|   IBIS file stm32l471_476_486_lqfp144.ibs
[IBIS ver]   4.2
[File name]   stm32l471_476_486_lqfp144.ibs
[File Rev]   4.0
[Date]   05-10-2018
[Source]   Data Created at STMicroelectronics
[Notes]   File originated from ELDO simulations.
[Disclaimer]  This information is for modeling purpose only and is
   not guaranteed.
   The information is subject to change without notice.
[Copyright]   Copyright 2018 STMicroelectronics Inc.
|   Component stm32l471_476_486_lqfp144
[Component] stm32l471_476_486_lqfp144
[Manufacturer] STMicroelectronics
[Package]
| variable   typ   min   max
R_pkg   0.0   0.0   0.0
L_pkg   0.0H   0.0H   0.0H
C_pkg   0.0F   0.0F   0.0F
[Pin]  signal_name   model_name   R_pin   L_pin   C_pin
1 PE2 io8prog2m25m50m120m_sudq_ft 187.6E-3 9.4E-9 267.9E-15
2 PE3 io8prog2m25m50m120m_sudq_ft 182.4E-3 9.1E-9 243.8E-15
3 PE4 io8prog2m25m50m120m_sudq_ft 177.6E-3 8.7E-9 221.3E-15
4 PE5 io8prog2m25m50m120m_sudq_ft 173.1E-3 8.4E-9 200.2E-15
5 PE6 io8prog2m25m50m120m_sudq_ft 168.9E-3 8.1E-9 180.5E-15
6 VBAT POWER 165.0E-3 7.8E-9 162.3E-15
7 PC13 io8prog2m25m50m120m_sudq_ft 161.5E-3 7.6E-9 145.6E-15
8 PC14-OSC32_IN io8prog2m25m50m120m_sudq_ft 158.2E-3 7.4E-9 130.3E-15
9 PC15-OSC32_OUT io8prog2m25m50m120m_sudq_ft 155.2E-3 7.2E-9 116.4E-15
10 PF0 io8prog2m25m50m120m_sudq_i2c_ft 152.6E-3 7.0E-9 104.1E-15
11 PF1 io8prog2m25m50m120m_sudq_i2c_ft 150.3E-3 6.8E-9 93.2E-15
12 PF2 io8prog2m25m50m120m_sudq_ft 148.2E-3 6.7E-9 83.7E-15
13 PF3 io8prog2m25m50m120m_sudq_ft 146.5E-3 6.5E-9 75.7E-15
14 PF4 io8prog2m25m50m120m_sudq_ft 145.1E-3 6.4E-9 69.1E-15
15 PF5 io8prog2m25m50m120m_sudq_ft 144.1E-3 6.4E-9 64.0E-15
16 VSS GND 143.3E-3 6.3E-9 60.4E-15
17 VDD POWER 142.8E-3 6.3E-9 58.2E-15
18 PF6 io8prog2m25m50m120m_sudq_ft 142.7E-3 6.3E-9 57.5E-15
19 PF7 io8prog2m25m50m120m_sudq_ft 142.7E-3 6.3E-9 57.5E-15
20 PF8 io8prog2m25m50m120m_sudq_ft 142.8E-3 6.3E-9 58.2E-15
21 PF9 io8prog2m25m50m120m_sudq_ft 143.3E-3 6.3E-9 60.4E-15
22 PF10 io8prog2m25m50m120m_sudq_ft 144.1E-3 6.4E-9 64.0E-15
23 PH0-OSC_IN io8prog2m25m50m120m_sudq_ft 145.1E-3 6.4E-9 69.1E-15
24 PH1-OSC_OUT io8prog2m25m50m120m_sudq_ft 146.5E-3 6.5E-9 75.7E-15
25 NRST ioreset_ft_v33 148.2E-3 6.7E-9 83.7E-15
26 PC0 io8prog2m25m50m120m_sudq_i2c_ft 150.3E-3 6.8E-9 93.2E-15
27 PC1 io8prog2m25m50m120m_sudq_i2c_ft 152.6E-3 7.0E-9 104.1E-15
28 PC2 io8prog2m25m50m120m_sudq_ft 155.2E-3 7.2E-9 116.4E-15
29 PC3 io8prog2m25m50m120m_sudq_ft 158.2E-3 7.4E-9 130.3E-15
30 VSSA GND 161.5E-3 7.6E-9 145.6E-15
31 VREF- GND 165.0E-3 7.8E-9 162.3E-15
32 VREF+ POWER 168.9E-3 8.1E-9 180.5E-15
33 VDDA POWER 173.1E-3 8.4E-9 200.2E-15
34 PA0 io8prog2m25m50m120m_sudq_ft 177.6E-3 8.7E-9 221.3E-15
35 PA1 io8prog2m25m50m120m_sudq_ft 182.4E-3 9.1E-9 243.8E-15
36 PA2 io8prog2m25m50m120m_sudq_ft 187.6E-3 9.4E-9 267.9E-15
37 PA3 io8prog2m25m50m120m_sudq_ft 187.6E-3 9.4E-9 267.9E-15
38 VSS GND 182.4E-3 9.1E-9 243.8E-15
39 VDD POWER 177.6E-3 8.7E-9 221.3E-15
40 PA4 io8prog2m25m50m120m_sudq_ft 173.1E-3 8.4E-9 200.2E-15
41 PA5 io8prog2m25m50m120m_sudq_ft 168.9E-3 8.1E-9 180.5E-15
42 PA6 io8prog2m25m50m120m_sudq_ft 165.0E-3 7.8E-9 162.3E-15
43 PA7 io8prog2m25m50m120m_sudq_ft 161.5E-3 7.6E-9 145.6E-15
44 PC4 io8prog2m25m50m120m_sudq_ft 158.2E-3 7.4E-9 130.3E-15
45 PC5 io8prog2m25m50m120m_sudq_ft 155.2E-3 7.2E-9 116.4E-15
46 PB0 io8prog2m25m50m120m_sudq_ft 152.6E-3 7.0E-9 104.1E-15
47 PB1 io8prog2m25m50m120m_sudq_ft 150.3E-3 6.8E-9 93.2E-15
48 PB2 io8prog2m25m50m120m_sudq_ft 148.2E-3 6.7E-9 83.7E-15
49 PF11 io8prog2m25m50m120m_sudq_ft 146.5E-3 6.5E-9 75.7E-15
50 PF12 io8prog2m25m50m120m_sudq_ft 145.1E-3 6.4E-9 69.1E-15
51 VSS GND 144.1E-3 6.4E-9 64.0E-15
52 VDD POWER 143.3E-3 6.3E-9 60.4E-15
53 PF13 io8prog2m25m50m120m_sudq_ft 142.8E-3 6.3E-9 58.2E-15
54 PF14 io8prog2m25m50m120m_sudq_ft 142.7E-3 6.3E-9 57.5E-15
55 PF15 io8prog2m25m50m120m_sudq_ft 142.7E-3 6.3E-9 57.5E-15
56 PG0 io8prog2m25m50m120m_sudq_ft 142.8E-3 6.3E-9 58.2E-15
57 PG1 io8prog2m25m50m120m_sudq_ft 143.3E-3 6.3E-9 60.4E-15
58 PE7 io8prog2m25m50m120m_sudq_ft 144.1E-3 6.4E-9 64.0E-15
59 PE8 io8prog2m25m50m120m_sudq_ft 145.1E-3 6.4E-9 69.1E-15
60 PE9 io8prog2m25m50m120m_sudq_ft 146.5E-3 6.5E-9 75.7E-15
61 VSS GND 148.2E-3 6.7E-9 83.7E-15
62 VDD POWER 150.3E-3 6.8E-9 93.2E-15
63 PE10 io8prog2m25m50m120m_sudq_ft 152.6E-3 7.0E-9 104.1E-15
64 PE11 io8prog2m25m50m120m_sudq_ft 155.2E-3 7.2E-9 116.4E-15
65 PE12 io8prog2m25m50m120m_sudq_ft 158.2E-3 7.4E-9 130.3E-15
66 PE13 io8prog2m25m50m120m_sudq_ft 161.5E-3 7.6E-9 145.6E-15
67 PE14 io8prog2m25m50m120m_sudq_ft 165.0E-3 7.8E-9 162.3E-15
68 PE15 io8prog2m25m50m120m_sudq_ft 168.9E-3 8.1E-9 180.5E-15
69 PB10 io8prog2m25m50m120m_sudq_i2c_ft 173.1E-3 8.4E-9 200.2E-15
70 PB11 io8prog2m25m50m120m_sudq_i2c_ft 177.6E-3 8.7E-9 221.3E-15
71 VSS GND 182.4E-3 9.1E-9 243.8E-15
72 VDD POWER 187.6E-3 9.4E-9 267.9E-15
73 PB12 io8w_swp_lcd4_ft 187.6E-3 9.4E-9 267.9E-15
74 PB13 io8prog2m25m50m120m_sudq_i2c_ft 182.4E-3 9.1E-9 243.8E-15
75 PB14 io8prog2m25m50m120m_sudq_i2c_ft 177.6E-3 8.7E-9 221.3E-15
76 PB15 io8prog2m25m50m120m_sudq_ft 173.1E-3 8.4E-9 200.2E-15
77 PD8 io8prog2m25m50m120m_sudq_ft 168.9E-3 8.1E-9 180.5E-15
78 PD9 io8prog2m25m50m120m_sudq_ft 165.0E-3 7.8E-9 162.3E-15
79 PD10 io8prog2m25m50m120m_sudq_ft 161.5E-3 7.6E-9 145.6E-15
80 PD11 io8prog2m25m50m120m_sudq_ft 158.2E-3 7.4E-9 130.3E-15
81 PD12 io8prog2m25m50m120m_sudq_ft 155.2E-3 7.2E-9 116.4E-15
82 PD13 io8prog2m25m50m120m_sudq_ft 152.6E-3 7.0E-9 104.1E-15
83 VSS GND 150.3E-3 6.8E-9 93.2E-15
84 VDD POWER 148.2E-3 6.7E-9 83.7E-15
85 PD14 io8prog2m25m50m120m_sudq_ft 146.5E-3 6.5E-9 75.7E-15
86 PD15 io8prog2m25m50m120m_sudq_ft 145.1E-3 6.4E-9 69.1E-15
87 PG2 io8prog2m25m50m120m_sudq_ft 144.1E-3 6.4E-9 64.0E-15
88 PG3 io8prog2m25m50m120m_sudq_ft 143.3E-3 6.3E-9 60.4E-15
89 PG4 io8prog2m25m50m120m_sudq_ft 142.8E-3 6.3E-9 58.2E-15
90 PG5 io8prog2m25m50m120m_sudq_ft 142.7E-3 6.3E-9 57.5E-15
91 PG6 io8prog2m25m50m120m_sudq_ft 142.7E-3 6.3E-9 57.5E-15
92 PG7 io8prog2m25m50m120m_sudq_i2c_ft 142.8E-3 6.3E-9 58.2E-15
93 PG8 io8prog2m25m50m120m_sudq_i2c_ft 143.3E-3 6.3E-9 60.4E-15
94 VSS GND 144.1E-3 6.4E-9 64.0E-15
95 VDDIO2 POWER 145.1E-3 6.4E-9 69.1E-15
96 PC6 io8prog2m25m50m120m_sudq_ft 146.5E-3 6.5E-9 75.7E-15
97 PC7 io8prog2m25m50m120m_sudq_ft 148.2E-3 6.7E-9 83.7E-15
98 PC8 io8prog2m25m50m120m_sudq_ft 150.3E-3 6.8E-9 93.2E-15
99 PC9 io8prog2m25m50m120m_sudq_ft 152.6E-3 7.0E-9 104.1E-15
100 PA8 io8prog2m25m50m120m_sudq_ft 155.2E-3 7.2E-9 116.4E-15
101 PA9 POWER 158.2E-3 7.4E-9 130.3E-15
102 PA10 io8usb_id_otg20_lcd4_ft_ms 161.5E-3 7.6E-9 145.6E-15
103 PA11 io8usblsfs_otg2 165.0E-3 7.8E-9 162.3E-15
104 PA12 io8usblsfs_otg2 168.9E-3 8.1E-9 180.5E-15
105 PA13 io8prog2m25m50m120m_sudq_ft 173.1E-3 8.4E-9 200.2E-15
106 VDDUSB/VDD POWER 177.6E-3 8.7E-9 221.3E-15
107 VSS GND 182.4E-3 9.1E-9 243.8E-15
108 VDD POWER 187.6E-3 9.4E-9 267.9E-15
109 PA14 io8prog2m25m50m120m_sudq_ft 187.6E-3 9.4E-9 267.9E-15
110 PA15 io8prog2m25m50m120m_sudq_ft 182.4E-3 9.1E-9 243.8E-15
111 PC10 io8prog2m25m50m120m_sudq_ft 177.6E-3 8.7E-9 221.3E-15
112 PC11 io8prog2m25m50m120m_sudq_ft 173.1E-3 8.4E-9 200.2E-15
113 PC12 io8prog2m25m50m120m_sudq_ft 168.9E-3 8.1E-9 180.5E-15
114 PD0 io8prog2m25m50m120m_sudq_ft 165.0E-3 7.8E-9 162.3E-15
115 PD1 io8prog2m25m50m120m_sudq_ft 161.5E-3 7.6E-9 145.6E-15
116 PD2 io8prog2m25m50m120m_sudq_ft 158.2E-3 7.4E-9 130.3E-15
117 PD3 io8prog2m25m50m120m_sudq_ft 155.2E-3 7.2E-9 116.4E-15
118 PD4 io8prog2m25m50m120m_sudq_ft 152.6E-3 7.0E-9 104.1E-15
119 PD5 io8prog2m25m50m120m_sudq_ft 150.3E-3 6.8E-9 93.2E-15
120 VSS GND 148.2E-3 6.7E-9 83.7E-15
121 VDD POWER 146.5E-3 6.5E-9 75.7E-15
122 PD6 io8prog2m25m50m120m_sudq_ft 145.1E-3 6.4E-9 69.1E-15
123 PD7 io8prog2m25m50m120m_sudq_ft 144.1E-3 6.4E-9 64.0E-15
124 PG9 io8prog2m25m50m120m_sudq_ft 143.3E-3 6.3E-9 60.4E-15
125 PG10 io8prog2m25m50m120m_sudq_ft 142.8E-3 6.3E-9 58.2E-15
126 PG11 io8prog2m25m50m120m_sudq_ft 142.7E-3 6.3E-9 57.5E-15
127 PG12 io8prog2m25m50m120m_sudq_ft 142.7E-3 6.3E-9 57.5E-15
128 PG13 io8prog2m25m50m120m_sudq_i2c_ft 142.8E-3 6.3E-9 58.2E-15
129 PG14 io8prog2m25m50m120m_sudq_i2c_ft 143.3E-3 6.3E-9 60.4E-15
130 VSS GND 144.1E-3 6.4E-9 64.0E-15
131 VDDIO2 POWER 145.1E-3 6.4E-9 69.1E-15
132 PG15 io8prog2m25m50m120m_sudq_ft 146.5E-3 6.5E-9 75.7E-15
133 PB3 io8prog2m25m50m120m_sudq_ft 148.2E-3 6.7E-9 83.7E-15
134 PB4 io8prog2m25m50m120m_sudq_ft 150.3E-3 6.8E-9 93.2E-15
135 PB5 io8prog2m25m50m120m_sudq_ft 152.6E-3 7.0E-9 104.1E-15
136 PB6 io8prog2m25m50m120m_sudq_i2c_ft 155.2E-3 7.2E-9 116.4E-15
137 PB7 io8prog2m25m50m120m_sudq_i2c_ft 158.2E-3 7.4E-9 130.3E-15
138 BOOT0 vpp_test_hv 161.5E-3 7.6E-9 145.6E-15
139 PB8 io8prog2m25m50m120m_sudq_i2c_ft 165.0E-3 7.8E-9 162.3E-15
140 PB9 io8prog2m25m50m120m_sudq_i2c_ft 168.9E-3 8.1E-9 180.5E-15
141 PE0 io8prog2m25m50m120m_sudq_ft 173.1E-3 8.4E-9 200.2E-15
142 PE1 io8prog2m25m50m120m_sudq_ft 177.6E-3 8.7E-9 221.3E-15
143 VSS GND 182.4E-3 9.1E-9 243.8E-15
144 VDD POWER 187.6E-3 9.4E-9 267.9E-15
[Model Selector] io8prog2m25m50m120m_sudq_ft
iols8p_sudq_ft_pd_lv  "IO low speed, PD=40kOhm - 1P8V"
iols8p_sudq_ft_pu_lv  "IO low speed, PU=40kOhm - 1P8V"
iols8p_sudq_ft_lv  "IO low speed - 1P8V"
iols8p_sudq_ft_pd  "IO low speed, PD=40kOhm - 3P3V"
iols8p_sudq_ft_pu  "IO low speed, PU=40kOhm - 3P3V"
iols8p_sudq_ft  "IO low speed - 3P3V"
iofs8p_sudq_ft_pd_lv  "IO full speed, PD=40kOhm - 1P8V"
iofs8p_sudq_ft_pu_lv  "IO full speed, PU=40kOhm - 1P8V"
iofs8p_sudq_ft_lv  "IO full speed - 1P8V"
iofs8p_sudq_ft_pd  "IO full speed, PD=40kOhm - 3P3V"
iofs8p_sudq_ft_pu  "IO full speed, PU=40kOhm - 3P3V"
iofs8p_sudq_ft  "IO full speed - 3P3V"
ioms8p_sudq_ft_pd_lv  "IO medium speed, PD=40kOhm - 1P8V"
ioms8p_sudq_ft_pu_lv  "IO medium speed, PU=40kOhm - 1P8V"
ioms8p_sudq_ft_lv  "IO medium speed - 1P8V"
ioms8p_sudq_ft_pd  "IO medium speed, PD=40kOhm - 3P3V"
ioms8p_sudq_ft_pu  "IO medium speed, PU=40kOhm - 3P3V"
ioms8p_sudq_ft  "IO medium speed - 3P3V"
iohs8p_sudq_ft_pd_lv  "IO high speed, PD=40kOhm - 1P8V"
iohs8p_sudq_ft_pu_lv  "IO high speed, PU=40kOhm - 1P8V"
iohs8p_sudq_ft_lv  "IO high speed - 1P8V"
iohs8p_sudq_ft_pd  "IO high speed, PD=40kOhm - 3P3V"
iohs8p_sudq_ft_pu  "IO high speed, PU=40kOhm - 3P3V"
iohs8p_sudq_ft  "IO high speed - 3P3V"
[Model Selector] io8prog2m25m50m120m_sudq_i2c_ft
io8prog_1v8_i2c_pd  "5V Tol GPIO 1.8V range i2c functionality with pull down"
io8prog_1v8_i2c_pu  "5V Tol GPIO 1.8V range i2c functionality with pull up"
io8prog_1v8_i2c  "5V Tol GPIO 1.8V range i2c functionality"
io8prog_3v3_i2c_pd  "5V Tol GPIO 3.3V range i2c functionality with pull down"
io8prog_3v3_i2c_pu  "5V Tol GPIO 3.3V range i2c functionality with pull up"
io8prog_3v3_i2c  "5V Tol GPIO 3.3V range i2c functionality"
io8ls_1v8_pd  "5V Tol GPIO 1.8V range with pd io low speed"
io8ls_1v8_pu  "5V Tol GPIO 1.8V range with pu io low speed"
io8ls_1v8  "5V Tol GPIO 1.8V range io low speed"
io8ls_3v3_pd  "5V Tol GPIO 3.3V range with pd io low speed"
io8ls_3v3_pu  "5V Tol GPIO 3.3V range with pu io low speed"
io8ls_3v3  "5V Tol GPIO 3.3V range io low speed"
io8fs_1v8_pd  "5V Tol GPIO 1.8V range with pd io full speed"
io8fs_1v8_pu  "5V Tol GPIO 1.8V range with pu io full speed"
io8fs_1v8  "5V Tol GPIO 1.8V range io full speed"
io8fs_3v3_pd  "5V Tol GPIO 3.3V range with pd io full speed"
io8fs_3v3_pu  "5V Tol GPIO 3.3V range with pu io full speed"
io8fs_3v3  "5V Tol GPIO 3.3V range io full speed"
io8ms_1v8_pd  "5V Tol GPIO 1.8V range with pd io medium speed"
io8ms_1v8_pu  "5V Tol GPIO 1.8V range with pu io medium speed"
io8ms_1v8  "5V Tol GPIO 1.8V range io medium speed"
io8ms_3v3_pd  "5V Tol GPIO 3.3V range with pd io medium speed"
io8ms_3v3_pu  "5V Tol GPIO 3.3V range with pu io medium speed"
io8ms_3v3  "5V Tol GPIO 3.3V range io medium speed"
io8hs_1v8_pd  "5V Tol GPIO 1.8V range with pd io high speed"
io8hs_1v8_pu  "5V Tol GPIO 1.8V range with pu io high speed"
io8hs_1v8  "5V Tol GPIO 1.8V range io high speed"
io8hs_3v3_pd  "5V Tol GPIO 3.3V range with pd io high speed"
io8hs_3v3_pu  "5V Tol GPIO 3.3V range with pu io high speed"
io8hs_3v3  "5V Tol GPIO 3.3V range io high speed"
[Model Selector] io8usb_id_otg20_lcd4_ft_ms
io8usbid_1v8_id_pu  "ID 1V8 range with pull up"
io8usbid_3v3_id_pu  "ID 3V3 range with pull up"
io8usbid_1v8_id  "ID 1V8 range"
io8usbid_3v3_id  "ID 3V3 range"
io8lsusbid_1v8_pd  "GPIO 1.8V range with pd io low speed"
io8lsusbid_1v8_pu  "GPIO 1.8V range with pu io low speed"
io8lsusbid_1v8  "GPIO 1.8V range io low speed"
io8lsusbid_3v3_pd  "GPIO 3.3V range with pd io low speed"
io8lsusbid_3v3_pu  "GPIO 3.3V range with pu io low speed"
io8lsusbid_3v3  "GPIO 3.3V range io low speed"
io8fsusbid_1v8_pd  "GPIO 1.8V range with pd io full speed"
io8fsusbid_1v8_pu  "GPIO 1.8V range with pu io full speed"
io8fsusbid_1v8  "GPIO 1.8V range io full speed"
io8fsusbid_3v3_pd  "GPIO 3.3V range with pd io full speed"
io8fsusbid_3v3_pu  "GPIO 3.3V range with pu io full speed"
io8fsusbid_3v3  "GPIO 3.3V range io full speed"
io8msusbid_1v8_pd  "GPIO 1.8V range with pd io medium speed"
io8msusbid_1v8_pu  "GPIO 1.8V range with pu io medium speed"
io8msusbid_1v8  "GPIO 1.8V range io medium speed"
io8msusbid_3v3_pd  "GPIO 3.3V range with pd io medium speed"
io8msusbid_3v3_pu  "GPIO 3.3V range with pu io medium speed"
io8msusbid_3v3  "GPIO 3.3V range io medium speed"
io8hsusbid_1v8_pd  "GPIO 1.8V range with pd io high speed"
io8hsusbid_1v8_pu  "GPIO 1.8V range with pu io high speed"
io8hsusbid_1v8  "GPIO 1.8V range io high speed"
io8hsusbid_3v3_pd  "GPIO 3.3V range with pd io high speed"
io8hsusbid_3v3_pu  "GPIO 3.3V range with pu io high speed"
io8hsusbid_3v3  "GPIO 3.3V range io high speed"
[Model Selector] io8usblsfs_otg2
usb_ls_pd  "USB Low Speed mode - Pull Down"
usb_ls_pu2  "USB Low Speed mode - Pull up 2"
usb_ls_pu  "USB Low Speed mode - Pull up"
usb_fs  "USB Low Speed mode"
usb_fs_pd  "USB Full Speed mode - Pull Down"
usb_fs_pu2  "USB Full Speed mode - Pull up 2"
usb_fs_pu  "USB Full Speed mode - Pull up"
[Model Selector] ioreset_ft_v33
ioreset_1v2_pu  "RESET 1.2V range with PU"
ioreset_1v2  "RESET 1.2V range"
ioreset_1v8_pu  "RESET 1.8V range with PU"
ioreset_1v8  "RESET 1.8V range"
ioreset_3v3_pu  "RESET 3.3V range with PU"
ioreset_3v3  "RESET 3.3V range"
[Model Selector] io8w_swp_lcd4_ft
io8w_swp_classc  "Class C swp functionality"
io8w_swp_classb  "Class B swp functionality"
io8lsw_1v8_pd  "GPIO 1.8V range with pd io low speed"
io8lsw_1v8_pu  "GPIO 1.8V range with pu io low speed"
io8lsw_1v8  "GPIO 1.8V range io low speed"
io8lsw_3v3_pd  "GPIO 3.3V range with pd io low speed"
io8lsw_3v3_pu  "GPIO 3.3V range with pu io low speed"
io8lsw_3v3  "GPIO 3.3V range io low speed"
io8fsw_1v8_pd  "GPIO 1.8V range with pd io full speed"
io8fsw_1v8_pu  "GPIO 1.8V range with pu io full speed"
io8fsw_1v8  "GPIO 1.8V range io full speed"
io8fsw_3v3_pd  "GPIO 3.3V range with pd io full speed"
io8fsw_3v3_pu  "GPIO 3.3V range with pu io full speed"
io8fsw_3v3  "GPIO 3.3V range io full speed"
io8msw_1v8_pd  "GPIO 1.8V range with pd io medium speed"
io8msw_1v8_pu  "GPIO 1.8V range with pu io medium speed"
io8msw_1v8  "GPIO 1.8V range io medium speed"
io8msw_3v3_pd  "GPIO 3.3V range with pd io medium speed"
io8msw_3v3_pu  "GPIO 3.3V range with pu io medium speed"
io8msw_3v3  "GPIO 3.3V range io medium speed"
io8hsw_1v8_pd  "GPIO 1.8V range with pd io high speed"
io8hsw_1v8_pu  "GPIO 1.8V range with pu io high speed"
io8hsw_1v8  "GPIO 1.8V range io high speed"
io8hsw_3v3_pd  "GPIO 3.3V range with pd io high speed"
io8hsw_3v3_pu  "GPIO 3.3V range with pu io high speed"
io8hsw_3v3  "GPIO 3.3V range io high speed"
[Model Selector] vpp_test_hv
vpp_1v8  "VPP with test functionality 1.8V range"
vpp_3v3  "VPP with test functionality 3.3V range"
| Models and submodels in the file (123): iols8p_sudq_ft_pd_lv (I/O), iols8p_sudq_ft_pu_lv (I/O), iols8p_sudq_ft_lv (I/O), iols8p_sudq_ft_pd (I/O), iols8p_sudq_ft_pu (I/O), iols8p_sudq_ft (I/O), iofs8p_sudq_ft_pd_lv (I/O), iofs8p_sudq_ft_pu_lv (I/O), iofs8p_sudq_ft_lv (I/O), iofs8p_sudq_ft_pd (I/O), iofs8p_sudq_ft_pu (I/O), iofs8p_sudq_ft (I/O), ioms8p_sudq_ft_pd_lv (I/O), ioms8p_sudq_ft_pu_lv (I/O), ioms8p_sudq_ft_lv (I/O), ioms8p_sudq_ft_pd (I/O), ioms8p_sudq_ft_pu (I/O), ioms8p_sudq_ft (I/O), iohs8p_sudq_ft_pd_lv (I/O), iohs8p_sudq_ft_pu_lv (I/O), iohs8p_sudq_ft_lv (I/O), iohs8p_sudq_ft_pd (I/O), iohs8p_sudq_ft_pu (I/O), iohs8p_sudq_ft (I/O), io8prog_1v8_i2c_pd (I/O), io8prog_1v8_i2c_pu (I/O), io8prog_1v8_i2c (I/O), io8prog_3v3_i2c_pd (I/O), io8prog_3v3_i2c_pu (I/O), io8prog_3v3_i2c (I/O), io8ls_1v8_pd (I/O), io8ls_1v8_pu (I/O), io8ls_1v8 (I/O), io8ls_3v3_pd (I/O), io8ls_3v3_pu (I/O), io8ls_3v3 (I/O), io8fs_1v8_pd (I/O), io8fs_1v8_pu (I/O), io8fs_1v8 (I/O), io8fs_3v3_pd (I/O), io8fs_3v3_pu (I/O), io8fs_3v3 (I/O), io8ms_1v8_pd (I/O), io8ms_1v8_pu (I/O), io8ms_1v8 (I/O), io8ms_3v3_pd (I/O), io8ms_3v3_pu (I/O), io8ms_3v3 (I/O), io8hs_1v8_pd (I/O), io8hs_1v8_pu (I/O), io8hs_1v8 (I/O), io8hs_3v3_pd (I/O), io8hs_3v3_pu (I/O), io8hs_3v3 (I/O), io8usbid_1v8_id_pu (Input), io8usbid_3v3_id_pu (Input), io8usbid_1v8_id (Input), io8usbid_3v3_id (Input), io8lsusbid_1v8_pd (I/O), io8lsusbid_1v8_pu (I/O), io8lsusbid_1v8 (I/O), io8lsusbid_3v3_pd (I/O), io8lsusbid_3v3_pu (I/O), io8lsusbid_3v3 (I/O), io8fsusbid_1v8_pd (I/O), io8fsusbid_1v8_pu (I/O), io8fsusbid_1v8 (I/O), io8fsusbid_3v3_pd (I/O), io8fsusbid_3v3_pu (I/O), io8fsusbid_3v3 (I/O), io8msusbid_1v8_pd (I/O), io8msusbid_1v8_pu (I/O), io8msusbid_1v8 (I/O), io8msusbid_3v3_pd (I/O), io8msusbid_3v3_pu (I/O), io8msusbid_3v3 (I/O), io8hsusbid_1v8_pd (I/O), io8hsusbid_1v8_pu (I/O), io8hsusbid_1v8 (I/O), io8hsusbid_3v3_pd (I/O)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
